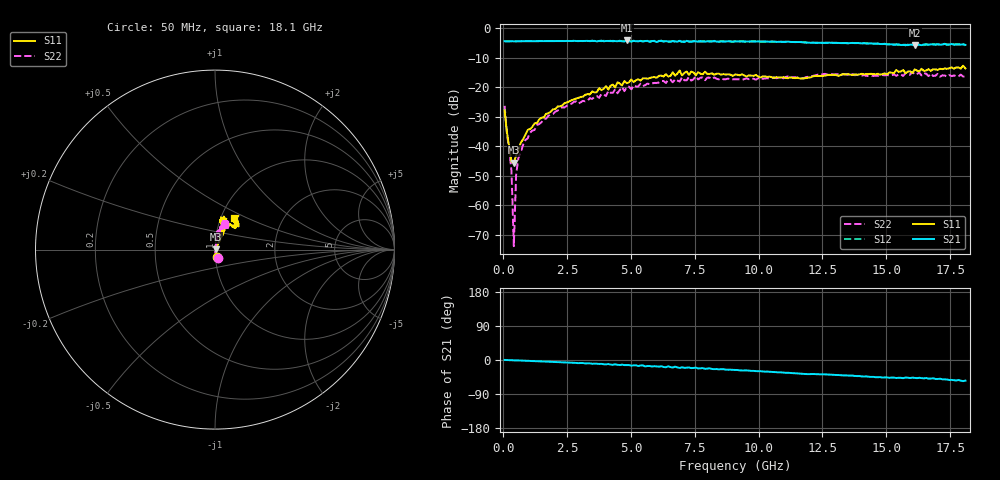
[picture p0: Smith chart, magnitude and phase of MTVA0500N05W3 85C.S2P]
! Network Analyzer HP8720D.06.14 Serial No. US36140669
!  8 Jul 2005  09:17:39
! Frequency  S11  S21  S12  S22
# HZ  S  DB R 50
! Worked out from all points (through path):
!   201 points, 50 MHz to 18.1 GHz, reference 50 ohm
!   highest |S21| = -4.22 dB at 4.833 GHz (marker M1); lowest = -5.8 dB at 16.11 GHz (marker M2)
!   group delay of S21, straight-line fit = 8.55 ps
!   lowest |S11| = -45.6 dB at 411 MHz (marker M3), VSWR 1.01, Z = 50.5 + j0.0709 ohm
!   |S11| at or under -10 dB: start of sweep to end of sweep
!   |S22| runs from -73.9 to -14.8 dB; largest |S21 - S12| = 0.027
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5e7  -27.90 -76.7  -4.46 0.2  -4.48 0.2  -26.36 -67.3
1.4025e8  -35.26 -68.3  -4.55 -0.1  -4.53 -0.2  -35.67 -82.5
3.2075e8  -45.29 -30.5  -4.46 -0.5  -4.49 -0.4  -48.63 -80.5
4.11e8  -45.56 7.7  -4.51 -0.9  -4.50 -1.0  -73.88 33.0
5.0125e8  -43.23 36.7  -4.49 -1.2  -4.48 -1.1  -49.70 76.2
5.915e8  -41.54 49.9  -4.47 -1.1  -4.50 -1.2  -43.94 86.9
8.6225e8  -36.16 57.4  -4.47 -1.8  -4.48 -1.9  -37.91 94.9
1.76475e9  -28.85 65.0  -4.41 -4.5  -4.41 -4.6  -29.73 76.9
3.1185e9  -23.26 65.9  -4.41 -8.0  -4.43 -8.4  -24.68 82.6
4.47225e9  -18.37 63.8  -4.49 -12.6  -4.35 -11.8  -22.11 83.7
4.83325e9  -18.69 73.3  -4.22 -13.4  -4.41 -14.1  -19.97 73.2
6.09675e9  -16.19 70.1  -4.43 -17.7  -4.35 -17.5  -18.47 74.8
6.7285e9  -16.16 77.3  -4.50 -17.6  -4.72 -18.5  -17.32 70.0
6.909e9  -14.40 75.1  -4.32 -20.9  -4.45 -19.4  -18.14 69.4
6.99925e9  -16.06 74.7  -4.61 -19.3  -4.72 -21.1  -16.67 70.9
7.17975e9  -14.74 79.3  -4.35 -20.4  -4.60 -19.5  -17.74 66.5
7.54075e9  -16.01 72.1  -4.53 -20.0  -4.40 -22.5  -16.33 74.8
9.075e9  -15.76 77.7  -4.53 -26.2  -4.51 -26.3  -17.35 66.8
1.21435e10  -16.34 67.5  -5.00 -36.9  -4.96 -37.0  -16.21 68.9
1.512175e10  -15.04 48.1  -5.55 -47.2  -5.39 -46.6  -16.11 71.7
1.61145e10  -14.03 49.9  -5.84 -47.1  -5.57 -47.0  -15.77 71.5
1.81e10  -13.70 58.5  -5.72 -54.5  -5.88 -55.5  -16.40 68.6
